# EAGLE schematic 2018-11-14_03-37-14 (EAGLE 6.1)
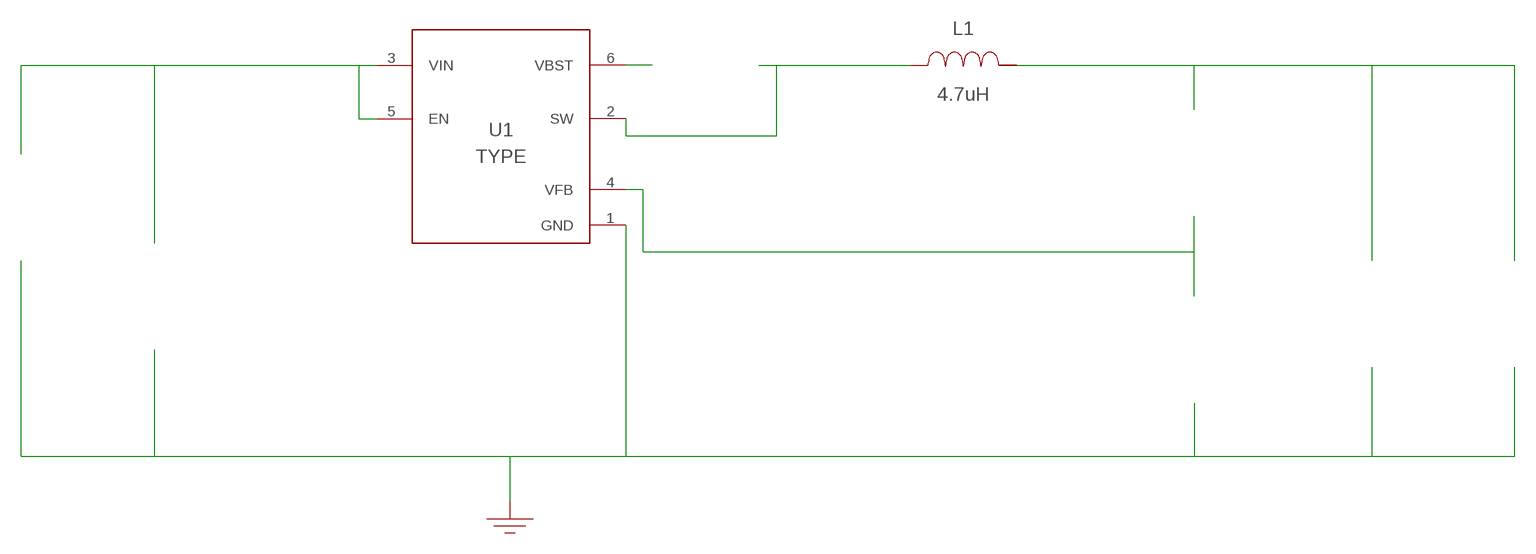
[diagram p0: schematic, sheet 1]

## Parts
CBST  100nF  C0603C104Z3VACTUC0603C104Z3VACTU  [0603]  (not placed on a sheet)
CIN  22uF  C2012X5R1V226M125ACC2012X5R1V226M125AC  [0805]  (not placed on a sheet)
COUT  47uF  C3216X5R1E476M160ACC3216X5R1E476M160AC  [1206]  (not placed on a sheet)
GND  WB_GND  WB_GNDWB_GND  [WB_GND]
IOUT  WB_CURRENT_LOAD  WB_CURRENT_LOADWB_CURRENT_LOAD  [WB_CURRENT_LOAD]  (not placed on a sheet)
L1  4.7uH  CDPH4D19FNP-4R7MCCDPH4D19FNP-4R7MC  [CDPH4D19F]
RFBB  10k  RC0201FR-0710KLRC0201FR-0710KL  [0201]  (not placed on a sheet)
RFBT  61.9k  CRCW040261K9FKEDCRCW040261K9FKED  [0402]  (not placed on a sheet)
U1  TPS561201DDCR  TPS561201DDCRTPS561201DDCR  [DDC0006A]
VIN  WB_BATTERY  WB_BATTERYWB_BATTERY  [WB_BATTERY]  (not placed on a sheet)

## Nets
0: Cin.2@2 Cout.2@2 GND.1 Iout.-@2 Rfbb.2@2 U1.1(GND) Vin.-@2
1: Cin.1@1 U1.3(VIN) U1.5(EN) Vin.+@1
2: Cbst.1@1 L1.1 U1.2(SW)
3: Rfbb.1@1 Rfbt.2@2 U1.4(VFB)
4: Cout.1@1 Iout.+@1 L1.2 Rfbt.1@1
5: Cbst.2@2 U1.6(VBST)
Unconnected: CBST.1 CBST.2 CIN.1 CIN.2 COUT.1 COUT.2 IOUT.1(+) IOUT.2(-) RFBB.1 RFBB.2 RFBT.1 RFBT.2 VIN.1(+) VIN.2(-)

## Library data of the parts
CBST = AcceleratedDesigns_Lib:C0603C104Z3VACTU; Cap: 1.0E-7; ESR: 0.0; IRMS: 0.0; Manufacturer_Name: Kemet; Manufacturer_Part_Number: C0603C104Z3VACTU; VDC: 25.0; Vendor: Kemet
CIN = AcceleratedDesigns_Lib:C2012X5R1V226M125AC; Cap: 2.2E-5; Datasheet_URL: https://product.tdk.com/en/search/capacitor/ceramic/mlcc/info?part%5Fno%3DC2012X5R1V226M125AC; ESR: 0.00205; IRMS: 4.55587; Manufacturer_Name: TDK; Manufacturer_Part_Number: C2012X5R1V226M125AC; VDC: 35.0; Vendor: TDK
COUT = AcceleratedDesigns_Lib:C3216X5R1E476M160AC; Cap_F: 0.000047; Manufacturer_Name: TDK; Manufacturer_Part_Number: C3216X5R1E476M160AC; MountType: SMT; RoHS: Y; VDC_V: 25
GND = AcceleratedDesigns_Lib:WB_GND; Manufacturer_Name: WB_GND; Manufacturer_Part_Number: WB_GND; PowerPortType: POWER_GROUND; Value: Value
IOUT = AcceleratedDesigns_Lib:WB_CURRENT_LOAD; Manufacturer_Name: WB_CURRENT_LOAD; Manufacturer_Part_Number: WB_CURRENT_LOAD; PowerPortType: POWER_GROUND; Value: Value
L1 = AcceleratedDesigns_Lib:CDPH4D19FNP-4R7MC; DCR: 0.038; IDC: 1.15; L: 4.7E-6; Manufacturer_Name: Sumida; Manufacturer_Part_Number: CDPH4D19FNP-4R7MC; Vendor: Sumida
RFBB = AcceleratedDesigns_Lib:RC0201FR-0710KL; Datasheet_URL: http://www.yageo.com/documents/recent/PYu%2DRC%5FGroup%5F51%5FRoHS%5FL%5F5.pdf; Manufacturer_Name: Yageo; Manufacturer_Part_Number: RC0201FR-0710KL; Power: 0.05; Resistance: 10000.0; Tolerance: 1.0; Vendor: Yageo America
RFBT = AcceleratedDesigns_Lib:CRCW040261K9FKED; Manufacturer_Name: Vishay-Dale; Manufacturer_Part_Number: CRCW040261K9FKED; Power: 0.063; Resistance: 61900.0; Tolerance: 1.0; Vendor: Vishay-Dale
U1 = AcceleratedDesigns_Lib:TPS561201DDCR; Manufacturer: Texas Instruments; Manufacturer_Name: Texas Instruments; Manufacturer_Part_Number: TPS561201DDCR; PartNumber: TPS561201DDCR; RefDes: RefDes; TYPE: TYPE; Value: Value
VIN = AcceleratedDesigns_Lib:WB_BATTERY; Manufacturer_Name: WB_BATTERY; Manufacturer_Part_Number: WB_BATTERY; PowerPortType: POWER_GROUND; Value: Value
